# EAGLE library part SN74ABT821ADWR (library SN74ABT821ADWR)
10-Bit Bus Interface Flip-Flops With 3-State Outputs Source: Datasheet
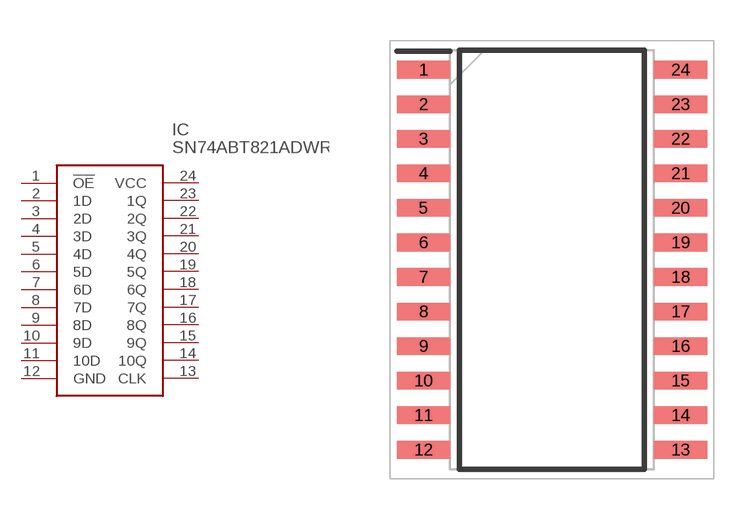
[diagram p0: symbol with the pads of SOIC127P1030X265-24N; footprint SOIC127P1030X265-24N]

Designator prefix IC

## SN74ABT821ADWR (Description: 10-Bit Bus Interface Flip-Flops With 3-State Outputs; Height: 2.65mm; Manufacturer_Name: Texas Instruments; Manufacturer_Part_Number: SN74ABT821ADWR; Mouser_Part_Number: 595-SN74ABT821ADWR; Mouser_Price-Stock: https://www.mouser.co.uk/ProductDetail/Texas-Instruments/SN74ABT821ADWR?qs=FM6NhYOeeBXxX%2Fnpl0SzFQ%3D%3D)  [SOIC127P1030X265-24N]
1  !OE
2  1D
3  2D
4  3D
5  4D
6  5D
7  6D
8  7D
9  8D
10  9D
11  10D
12  GND
13  CLK
14  10Q
15  9Q
16  8Q
17  7Q
18  6Q
19  5Q
20  4Q
21  3Q
22  2Q
23  1Q
24  VCC

## Footprint SOIC127P1030X265-24N (pad centres in mm)
DW (R-PDSO-G24)
smd 1.95 x 0.65: 1 -4.725,6.985; 2 -4.725,5.715; 3 -4.725,4.445; 4 -4.725,3.175; 5 -4.725,1.905; 6 -4.725,0.635; 7 -4.725,-0.635; 8 -4.725,-1.905; 9 -4.725,-3.175; 10 -4.725,-4.445; 11 -4.725,-5.715; 12 -4.725,-6.985; 13 4.725,-6.985; 14 4.725,-5.715; 15 4.725,-4.445; 16 4.725,-3.175; 17 4.725,-1.905; 18 4.725,-0.635; 19 4.725,0.635; 20 4.725,1.905; 21 4.725,3.175; 22 4.725,4.445; 23 4.725,5.715; 24 4.725,6.985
